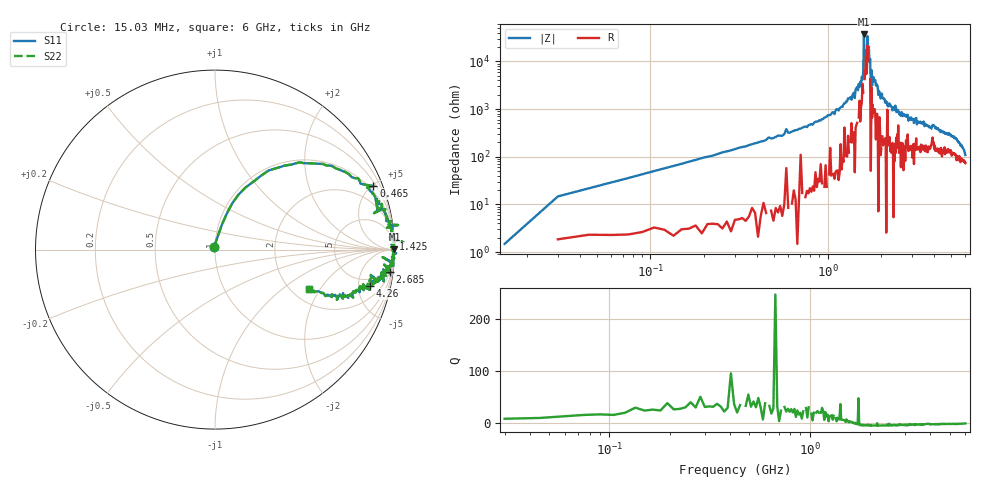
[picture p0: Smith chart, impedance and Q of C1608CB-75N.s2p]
!	Network	Analyzer	HP8753E.07.74:	Oct	30	2002	Serial	No.	JP38451487
!	Hewlett-Packard
!	28	Aug	2009	8:23:50
!	Frequency	S11	S21	S12	S22
#	HZ	S	RI	R	50
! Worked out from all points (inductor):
!   400 points, 15.03 MHz to 6 GHz, reference 50 ohm
!   read as one part in series: L = 76.2 nH near 45.03 MHz
!   highest |Z| = 36.8 kohm at 1.605 GHz (marker M1)
!   self-resonance near 1.65 GHz
!   S11 on the Smith chart (normalised r, x): 15.03 MHz: 0.99, +0.03; 465 MHz: 0.68, +5.09; 1.425 GHz: 2, +34; 2.685 GHz: 2, -16; 4.26 GHz: 3.60, -6.78; 6 GHz: 2.47, -1.60
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1.502992e7  -0.00601 0.0127  1.01 -0.0127  1.01 -0.0127  -0.00601 0.0127
3.002985e7  0.038 0.138  0.962 -0.138  0.962 -0.138  0.038 0.138
9.002955e7  0.171 0.347  0.829 -0.347  0.829 -0.347  0.171 0.347
4.650277e8  0.883 0.354  0.117 -0.354  0.117 -0.354  0.883 0.354
1.020025e9  0.975 0.129  0.0246 -0.129  0.0246 -0.129  0.975 0.129
1.425023e9  0.995 0.0583  0.00504 -0.0583  0.00504 -0.0583  0.995 0.0583
1.575022e9  0.981 0.0135  0.0189 -0.0135  0.0189 -0.0135  0.981 0.0135
1.605022e9  1 0.000915  -0.00256 -0.000915  -0.00256 -0.000915  1 0.000915
1.635022e9  0.987 0.00439  0.0128 -0.00439  0.0128 -0.00439  0.987 0.00439
1.650022e9  0.995 0.00354  0.00452 -0.00354  0.00452 -0.00354  0.995 0.00354
1.665022e9  0.99 -0.00879  0.0102 0.00879  0.0102 0.00879  0.99 -0.00879
1.680022e9  0.998 -0.00226  0.00186 0.00226  0.00186 0.00226  0.998 -0.00226
1.710021e9  0.998 -0.00421  0.00247 0.00421  0.00247 0.00421  0.998 -0.00421
1.755021e9  0.997 0.0416  0.00262 -0.0416  0.00262 -0.0416  0.997 0.0416
1.770021e9  0.993 -0.0135  0.00668 0.0135  0.00668 0.0135  0.993 -0.0135
2.01002e9  0.993 -0.051  0.00653 0.051  0.00653 0.051  0.993 -0.051
2.685017e9  0.976 -0.123  0.0239 0.123  0.0239 0.123  0.976 -0.123
3.015015e9  0.954 -0.146  0.0456 0.146  0.0456 0.146  0.954 -0.146
4.00501e9  0.893 -0.18  0.107 0.18  0.107 0.18  0.893 -0.18
4.260009e9  0.863 -0.202  0.137 0.202  0.137 0.202  0.863 -0.202
5.010005e9  0.804 -0.223  0.196 0.223  0.196 0.223  0.804 -0.223
6e9  0.524 -0.219  0.476 0.219  0.476 0.219  0.524 -0.219
